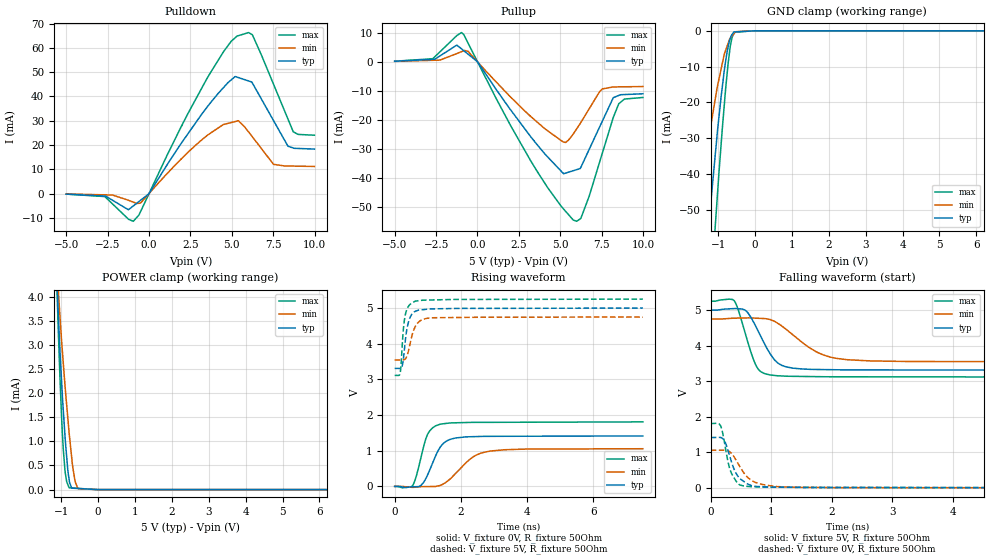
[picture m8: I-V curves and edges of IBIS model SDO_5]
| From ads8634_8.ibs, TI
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|   SDO_5   5V digital 3-state Model
[Model] SDO_5   | 5V digital 3-state
Model_type 3-state
Polarity   Non-Inverting
Vmeas = 2.5
Vref = 2.5
Cref = 15pF
Rref = 50
|   typ   min   max
|   (nom PVT)   (Fast PVT)   (slow PVT)
|BUFFER OUTPUT TURNED HIGH
|C_comp from L-C Tank method(L=1nH)
|Resonant Frequency(Hz)   4.48G   4.89G   4.07G
|C_comp   1.26497E-12   1.06189E-12   1.52785E-12
|BUFFER OUTPUT LOW
|C_comp from L-C Tank method(L=1nH)
|Resonant Frequency(Hz)   4.37G   4.81G   4.04G
|C_comp   1.32459E-12   1.09668E-12   1.55626E-12
|BUFFER HIGH Z STATE
|C_comp from L-C Tank method(L=1nH)
|Resonant Frequency(Hz)   4.09G   4.48G   3.90G
C_comp   1.51384E-12   1.26497E-12   1.66756E-12
| Where   nom PVT is  Nominal Process, 5V, 25C
|   Fast PVT is Strong Process, 4.5V, -40C
|   Slow PVT is Weak Process, 5.5V, 85C
|C_comp - from L-C Tank method, L = 1nH, peak frequency
[Voltage Range]   5   4.75   5.25
[Temperature Range]   27   125   -40
[Pullup Reference]   5   4.75   5.25
[Pulldown Reference]   0   0   0
[Power Clamp Reference]   5   4.75   5.25
[GND Clamp Reference]   0   0   0
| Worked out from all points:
|   slope of the pulldown table from 0 to 0.75 V, typ, clamps not added: 92 ohm
|   slope of the pullup table from 0 to 0.75 V, typ, clamps not added: 119 ohm
|   GND clamp passes 1 mA (typ) near -0.62 V on its own axis
|   POWER clamp passes 1 mA (typ) near -0.89 V on its own axis
|   falling waveform, V_fixture 5V, R_fixture 50Ohm: 20-80 % time 325ps typ, 587ps min, 234ps max; typ from 5 V to 3.31 V
|   rising waveform, V_fixture 0V, R_fixture 50Ohm: 20-80 % time 424ps typ, 721ps min, 313ps max; typ from 0.002 V to 1.42 V
|   rising waveform, V_fixture 5V, R_fixture 50Ohm: 20-80 % time 162ps typ, 225ps min, 123ps max; typ from 3.31 V to 5 V
|   falling waveform, V_fixture 0V, R_fixture 50Ohm: 20-80 % time 199ps typ, 277ps min, 149ps max; typ from 1.42 V to 0.003 V
[Pulldown]
|   Voltage   I(typ)   I(min)   I(max)
-5V       -231.5uA   -154.2uA   -236.1uA
-2.671V   -1.028mA   -545.3uA   -1.246mA
-953.8mV  -5.126mA   -3.534mA   -11.44mA
-9.578mV  -106.5uA   -73.93uA   -141.8uA
2.324V    24.4mA     16.8mA     32.66mA
4.471V    43.49mA    28.38mA    58.17mA
5.388V    47.79mA    30.01mA    65.02mA
6.007V    46.39mA    25.39mA    66.32mA
6.253V    45.35mA    23.24mA    65.16mA
7.511V    30.1mA     12.06mA    45.08mA
8.702V    18.78mA    11.31mA    25.48mA
9.985V    18.32mA    11.16mA    24.03mA
[GND Clamp]
|   Voltage   I(typ)   I(min)   I(max)
-5V       -576.4mA   -401.2mA   -708.5mA
-1.671V   -107mA     -62.05mA   -151.4mA
-1.518V   -87.19mA   -49.42mA   -126.2mA
-1.248V   -53.68mA   -29.75mA   -81.61mA
-1.101V   -37.4mA    -20.59mA   -58.33mA
-1.023V   -28.8mA    -15.8mA    -46.71mA
-891.4mV  -16.18mA   -9.422mA   -28.13mA
-814mV    -9.761mA   -6.01mA    -18.52mA
-727.9mV  -4.499mA   -3.504mA   -9.126mA
-672.4mV  -2.242mA   -2.105mA   -4.539mA
-571.3mV  -319.2uA   -844.6uA   -713.2uA
9.985V    0A         0A         0A
[Pullup]
|   Voltage   I(typ)   I(min)   I(max)
-5V       186.9uA    141uA      205.3uA
-2.703V   833uA      520.6uA    1.055mA
-1.248V   5.753mA    2.838mA    9.019mA
-829.2mV  3.835mA    3.81mA     9.37mA
-9.578mV  82.51uA    60.75uA    109.7uA
3.192V    -25.6mA    -18.7mA    -33.87mA
5.169V    -38.33mA   -27.57mA   -50.47mA
5.984V    -37.1mA    -23.08mA   -54.87mA
6.244V    -36.23mA   -20.83mA   -53.79mA
7.534V    -20.45mA   -9.339mA   -31.49mA
8.53V     -11.57mA   -8.625mA   -14.42mA
9.985V    -11mA      -8.507mA   -12.27mA
[POWER Clamp]
|   Voltage   I(typ)   I(min)   I(max)
-5V       90.84mA    71.45mA    115.5mA
-1.237V   6.671mA    6.389mA    7.28mA
-1.089V   3.814mA    4.304mA    3.534mA
-1.061V   3.333mA    3.912mA    2.911mA
-987.9mV  2.223mA    3.067mA    1.472mA
-941.7mV  1.618mA    2.606mA    816.3uA
-891.4mV  1.041mA    2.106mA    355.2uA
-786.2mV  210.5uA    1.184mA    38.56uA
-718.2mV  30.24uA    683.2uA    35.08uA
-624.6mV  26.25uA    172.4uA    30.28uA
-532.4mV  22.31uA    18.56uA    25.56uA
9.985V    0A         0A         0A
[Ramp]
R_load = 50
|   typ   min   max
dV/dt_r   0.847964/4.24064e-010   0.63281/7.18598e-010   1.08519/3.12541e-010
dV/dt_f   1.01404/3.23247e-010  0.721416/5.83655e-010   1.28164/2.33742e-010
[Falling Waveform]
V_fixture = 5V
V_fixture_min = 4.75V
V_fixture_max = 5.25V
R_fixture = 50Ohm
C_fixture = 0F
|   Time   V(typ)   V(min)   V(max)
0s        4.999V     4.749V     5.25V
387.9ps   5.043V     4.773V     5.266V
570ps     4.998V     4.78V      4.353V
746ps     4.54V      4.773V     3.454V
830.4ps   4.251V     4.767V     3.266V
979.5ps   3.779V     4.736V     3.177V
1.249ns   3.403V     4.457V     3.141V
1.766ns   3.33V      3.81V      3.129V
2.241ns   3.319V     3.608V     3.125V
7.5ns     3.309V     3.546V     3.114V
[Rising Waveform]
V_fixture = 0V
V_fixture_min = 0V
V_fixture_max = 0V
R_fixture = 50Ohm
C_fixture = 0F
|   Time   V(typ)   V(min)   V(max)
0s        2.499mV    2.516mV    894.2uV
538.9ps   -8.713mV   -25.72mV   22.95mV
655.9ps   -6.767mV   -17.73mV   298.8mV
791.9ps   28.68mV    -7.167mV   801.3mV
985.3ps   306.1mV    -3.493mV   1.443V
1.368ns   1.088V     26.27mV    1.743V
1.813ns   1.353V     338.4mV    1.784V
2.369ns   1.396V     828.2mV    1.796V
2.877ns   1.405V     989.4mV    1.797V
7.5ns     1.416V     1.057V     1.81V
[Rising Waveform]
V_fixture = 5V
V_fixture_min = 4.75V
V_fixture_max = 5.25V
R_fixture = 50Ohm
C_fixture = 0F
|   Time   V(typ)   V(min)   V(max)
0s        3.309V     3.546V     3.114V
167.7ps   3.308V     3.545V     3.185V
221.3ps   3.359V     3.545V     3.85V
264.3ps   3.58V      3.547V     4.419V
336.9ps   4.201V     3.588V     4.872V
447.4ps   4.696V     3.923V     5.087V
630.9ps   4.911V     4.496V     5.195V
854.2ps   4.954V     4.684V     5.22V
1.182ns   4.976V     4.728V     5.228V
7.5ns     4.999V     4.748V     5.25V
[Falling Waveform]
|Gnd
V_fixture = 0V
V_fixture_min = 0V
V_fixture_max = 0V
R_fixture = 50Ohm
C_fixture = 0F
|   Time   V(typ)   V(min)   V(max)
0s        1.416V     1.058V     1.81V
161.4ps   1.419V     1.059V     1.752V
235ps     1.299V     1.059V     1.202V
286.9ps   1.047V     1.039V     724.3mV
332.2ps   794.3mV    989.2mV    455.7mV
442.2ps   345.7mV    712.5mV    137.5mV
556.9ps   169.9mV    401.8mV    49.27mV
810ps     35.13mV    112.2mV    27.75mV
1.394ns   15.03mV    16.6mV     17.73mV
7.5ns     2.535mV    2.822mV    895.2uV
